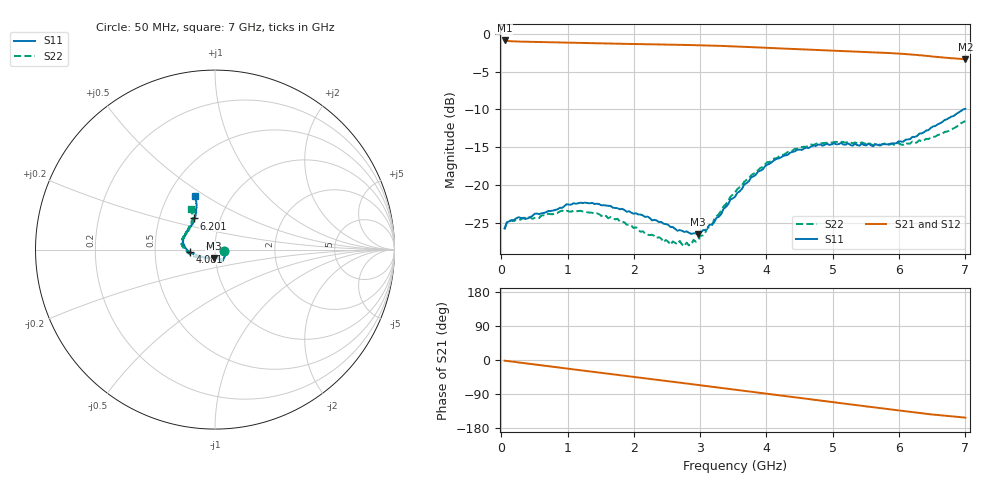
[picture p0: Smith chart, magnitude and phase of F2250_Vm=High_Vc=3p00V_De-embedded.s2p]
! Integrated Device Technology
! Corporate Headquarters
! 6024 Silver Creek Valley Road
! San Jose, CA 95138  USA
! Phone:  1-408-284-8200
! Toll Free:  1-800-223-1366
! Webpage:  http://www.idt.com/
! Timing and RF Division
! 515 Groton Road, Suite 102
! Westford, MA 01886-6024
! Device:  F2250
! Description: Voltage Variable RF Attenuator
! Frequency:  50.0 -  6000.00 MHz
! Package:  3x3 mm Thin QFN Plastic Package: 16 pin
! Ports:  2 RF, 3 DC
!  Pin  1  = GND
!  Pin  2  = NC
!  Pin  3  = RF1  = Port 1
!  Pin  4  = NC
!  Pin  5  = GND
!  Pin  6  = GND
!  Pin  7  = GND
!  Pin  8  = GND
!  Pin  9  = NC
!  Pin 10  = RF2  = Port 2
!  Pin 11  = NC
!  Pin 12  = GND
!  Pin 13  = GND
!  Pin 14  = VCNTRL
!  Pin 15  = VDD
!  Pin 16  = VMODE
! Vcntrl:  3.000 Volts
! Vmode:  +3.300 Volts
! Vdd:  +3.30  Volts
! Current:  1.315 mA
! Data:  The device was measured on a the F2250 evaluation board which has
!  individual transmission lines to the RF pins.  Data was collected
!  using a calibrated network analyzer.  The evaluation board was
!  de-embedded using a TRL calibration technique.
!  The reference plane is the edge of the package pin.
! Misc:  SN 10
!  Action Tracker AT0258
! Date Measured:  2014-11-26
! Date:  2015-10-15  MJV
! Note:
!  Integrated Device Technology supplies this data as a sample of measured
!  data at the package pin for this product.  Your particular data for this
!  product may vary.
!  Data was taken at 25 degrees C.
!  Integrated Device Technology reserves the right to change this data at anytime.
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# GHz S dB R 50
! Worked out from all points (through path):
!   201 points, 50 MHz to 7 GHz, reference 50 ohm
!   highest |S21| = -0.89 dB at 50 MHz (marker M1); lowest = -3.4 dB at 7 GHz (marker M2)
!   group delay of S21, straight-line fit = 61.2 ps
!   lowest |S11| = -26.5 dB at 2.969 GHz (marker M3), VSWR 1.10, Z = 49.1 - j4.62 ohm
!   |S11| at or under -10 dB: start of sweep to 6.968 GHz
!   |S22| runs from -28.0 to -11.5 dB; largest |S21 - S12| = 0.002
!   S11 on the Smith chart (normalised r, x): 50 MHz: 1.11, -0.02; 4.081 GHz: 0.75, -0.02; 6.201 GHz: 0.75, +0.27; 7 GHz: 0.68, +0.45
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0.05  -25.69 -10.8  -0.89 -1.8  -0.89 -1.8  -25.84 -11.0
0.1195  -24.77 -10.2  -0.99 -3.2  -0.98 -3.2  -24.70 -8.8
0.57125  -23.84 -31.3  -1.10 -13.3  -1.10 -13.3  -24.33 -31.4
0.91875  -23.00 -50.1  -1.17 -21.0  -1.17 -21.1  -23.36 -51.0
1.2315  -22.36 -57.9  -1.24 -27.9  -1.24 -27.9  -23.47 -61.5
1.75275  -23.04 -64.8  -1.33 -39.1  -1.33 -39.1  -24.42 -67.8
2.37825  -24.87 -64.5  -1.42 -52.8  -1.42 -52.8  -26.86 -66.7
2.552  -25.51 -69.4  -1.44 -56.7  -1.45 -56.7  -27.86 -73.0
2.691  -25.92 -77.5  -1.47 -59.8  -1.47 -59.8  -27.36 -80.8
2.7605  -26.17 -79.7  -1.48 -61.3  -1.49 -61.3  -28.05 -85.2
2.969  -26.49 -97.8  -1.52 -66.0  -1.52 -66.0  -27.28 -104.8
3.1775  -25.21 -120.8  -1.57 -70.7  -1.57 -70.7  -25.25 -126.7
3.525  -21.53 -152.8  -1.68 -78.5  -1.68 -78.6  -20.97 -148.7
3.76825  -18.97 -164.8  -1.77 -84.0  -1.77 -84.0  -18.70 -159.6
4.081  -16.95 -175.7  -1.90 -91.0  -1.90 -91.0  -16.72 -171.4
4.4285  -15.54 176.0  -2.03 -98.6  -2.04 -98.7  -15.19 178.7
4.7065  -14.76 169.1  -2.13 -104.8  -2.13 -104.8  -14.68 173.0
5.054  -14.60 160.9  -2.26 -112.5  -2.25 -112.5  -14.27 166.0
5.85325  -14.57 135.1  -2.56 -130.0  -2.56 -130.1  -14.67 147.3
6.20075  -13.62 123.6  -2.77 -137.7  -2.77 -137.8  -14.24 138.3
6.54825  -12.18 115.6  -3.04 -144.7  -3.04 -144.9  -13.58 126.9
7  -9.91 110.7  -3.37 -152.1  -3.37 -152.2  -11.54 120.7
